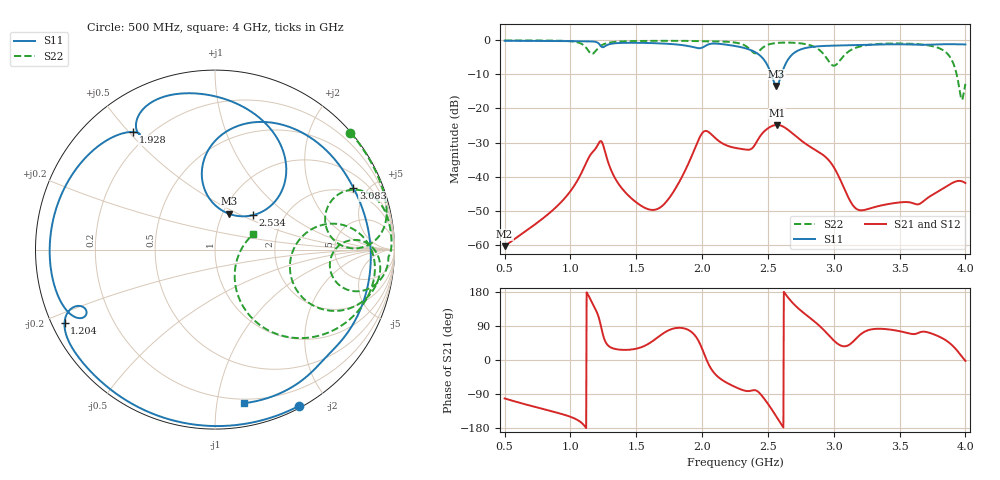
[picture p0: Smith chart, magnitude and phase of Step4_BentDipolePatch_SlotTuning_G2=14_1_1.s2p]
! TOUCHSTONE file generated by CST MICROWAVE STUDIO
! Date and time: Wed May 20 12:18:26 2020
! Project name: DualBand_DualMode_Antenna_FD_SteppedDesign.cst
! Parameters = {FPL=20; FPW=20; L=50; ST=10; SW=30; W=52; WF=7; ext=10; gap=1; inset=13}
! Header version: 2015
! Port assignment regex: !\s*Touchstone port\s*([0-9]+)\s*=\s*CST MWS port\s*([0-9]+)\s*\(\"(.*)\"\)(\s*mode\s*([0-9]+))?.*
! Touchstone port assignment:
! Touchstone port 1 = CST MWS port 1 ("")
! Touchstone port 2 = CST MWS port 2 ("")
# GHz S MA R 50
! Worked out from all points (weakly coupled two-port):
!   1006 points, 500 MHz to 4 GHz, reference 50 ohm
!   highest |S21| = -24.83 dB at 2.568 GHz (marker M1); lowest = -60.4 dB at 500 MHz (marker M2)
!   lowest |S11| = -13.4 dB at 2.565 GHz (marker M3), VSWR 1.55, Z = 53.5 + j22.4 ohm
!   |S11| at or under -10 dB: 2.526 GHz to 2.603 GHz (77.27 MHz wide, 3.01 % of centre)
!   |S22| runs from -17.4 to 0.0 dB; largest |S21 - S12| = 1.9e-05
!   S11 on the Smith chart (normalised r, x): 500 MHz: 0.02, -1.68; 1.204 GHz: 0.04, -0.23; 1.928 GHz: 0.14, +0.51; 2.534 GHz: 1.40, +0.59; 3.083 GHz: 1.68, +4.03; 4 GHz: 0.17, -1.19
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0.5  0.9886 -61.6  0.0009509 -101.4  0.0009509 -101.4  0.9967 40.8
0.794  0.9814 -97.9  0.00246 -129.5  0.002459 -129.5  0.9948 21.8
1.0845  0.9703 -134.6  0.0114 -165.7  0.0114 -165.8  0.8891 3.1
1.2035  0.9319 -154.1  0.02819 123.6  0.02819 123.6  0.747 24.0
1.431  0.9207 -173.2  0.005491 26.8  0.005495 26.8  0.9709 12.7
1.669  0.9046 156.5  0.0034 61.4  0.003401 61.4  0.984 6.0
1.928  0.7993 124.9  0.02152 71.4  0.02152 71.4  0.9797 -0.4
2.026  0.8313 121.9  0.04682 7.1  0.04682 7.1  0.9674 -2.6
2.25  0.8266 82.6  0.0264 -71.0  0.0264 -71.0  0.9289 -11.1
2.4005  0.6759 56.3  0.02915 -79.7  0.02915 -79.7  0.6461 -8.0
2.5335  0.2867 42.1  0.05551 -132.7  0.0555 -132.7  0.8977 -0.9
2.565  0.2142 68.8  0.05733 -149.9  0.05733 -149.8  0.9151 -3.2
2.5685  0.2151 73.0  0.05736 -151.8  0.05736 -151.8  0.9164 -3.4
2.6525  0.5219 96.0  0.04864 165.1  0.04864 165.1  0.9273 -8.9
2.8345  0.801 58.1  0.02637 107.0  0.02637 107.0  0.831 -22.7
2.9815  0.8355 36.5  0.0156 58.1  0.0156 58.1  0.4435 -18.2
3.083  0.8445 24.0  0.006464 36.2  0.006464 36.2  0.6132 12.9
3.188  0.8565 11.8  0.003241 62.7  0.003245 62.7  0.8024 6.9
3.419  0.8752 -14.9  0.003965 80.6  0.003965 80.7  0.8979 -7.2
3.853  0.8785 -62.3  0.007108 51.6  0.007107 51.6  0.6655 -47.7
3.9685  0.8742 -75.7  0.008578 11.2  0.008579 11.2  0.1387 -31.4
4  0.8709 -79.4  0.008033 -2.4  0.008035 -2.4  0.2298 21.9
